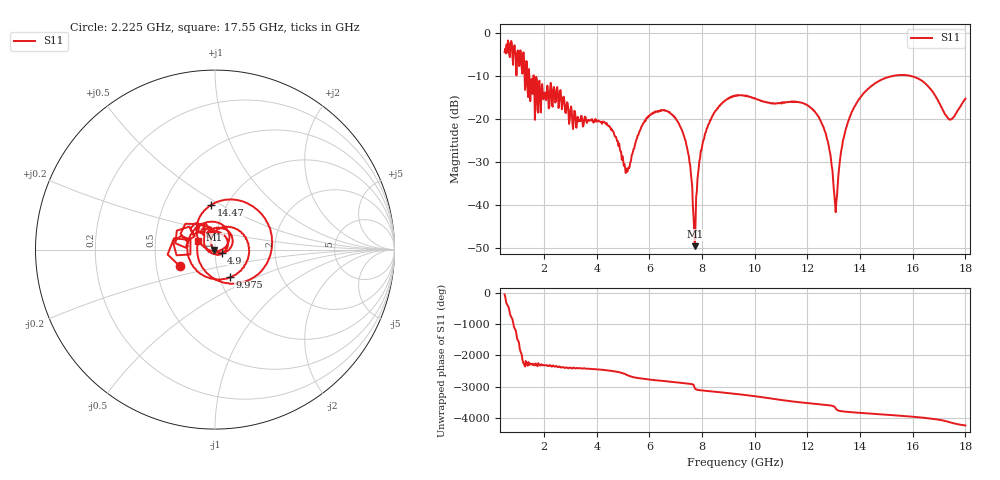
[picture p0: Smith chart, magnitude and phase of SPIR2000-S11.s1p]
!Keysight Technologies,P9374A,MY57211922,A.15.40.13
!Date: Sunday, October 20, 2024 14:33:54
!Correction: S11(C  1-Port  )
!S1P File: Measurement: S11:
# Hz S  dB  R 50
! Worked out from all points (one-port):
!   701 points, 500 MHz to 18 GHz, reference 50 ohm
!   lowest |S11| = -49.6 dB at 7.725 GHz (marker M1), VSWR 1.01, Z = 49.7 - j0.0458 ohm
!   |S11| at or under -10 dB: 1.439 GHz to 1.599 GHz (159.3 MHz wide, 10.5 % of centre); 1.603 GHz to 15.19 GHz (13.59 GHz wide, 162 % of centre); 15.98 GHz to end of sweep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
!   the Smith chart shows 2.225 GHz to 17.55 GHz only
!   S11 on the Smith chart (normalised r, x): 2.225 GHz: 0.66, -0.13; 4.9 GHz: 1.08, -0.04; 9.975 GHz: 1.12, -0.36; 14.47 GHz: 0.85, +0.45; 17.55 GHz: 0.82, +0.08
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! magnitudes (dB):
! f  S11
! 500 MHz  -4.4
! 1.175 GHz  -9.4
! 1.7 GHz  -10.1
! 2.225 GHz  -13.3
! 2.7 GHz  -16.4
! 3.15 GHz  -18.0
! 4.4 GHz  -21.4
! 4.875 GHz  -26.9
! 4.9 GHz  -27.5
! 5.175 GHz  -32.0
! 5.95 GHz  -19.3
! 7.075 GHz  -20.6
! 7.475 GHz  -28.0
! 7.725 GHz  -49.6
! 7.9 GHz  -29.6
! 8.175 GHz  -22.1
! 9.25 GHz  -14.4
! 9.975 GHz  -15.2
! 11.45 GHz  -16.0
! 12.55 GHz  -21.0
! 12.82 GHz  -26.8
! 13.07 GHz  -41.6
! 13.32 GHz  -26.1
! 13.62 GHz  -19.2
! 14.47 GHz  -12.0
! 15.82 GHz  -9.8
! 17.55 GHz  -19.5
! 18 GHz  -15.2
